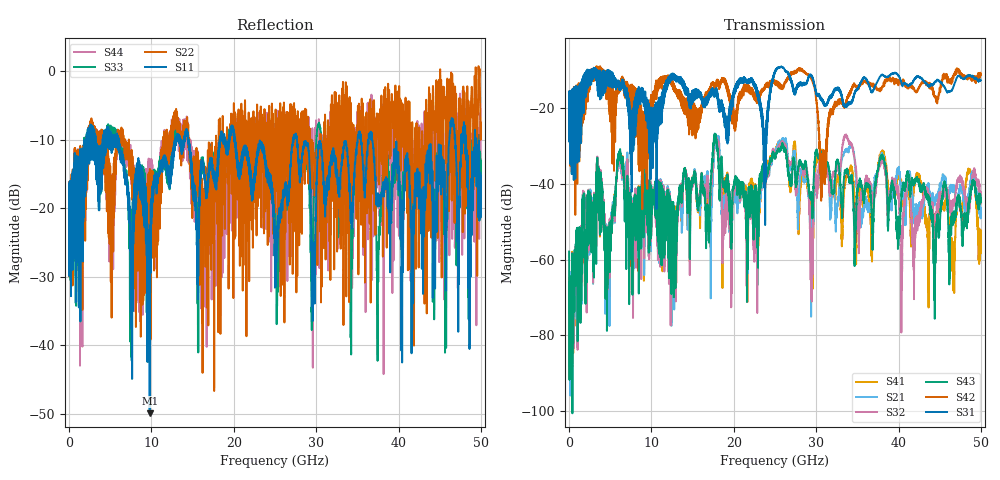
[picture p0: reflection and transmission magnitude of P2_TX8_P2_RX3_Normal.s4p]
!Keysight Technologies,N5225B,MY57041031,A.13.20.10
!Date: Friday, May 31, 2019 11:31:29
!Correction: S11(Full 4 Port(1,2,3,4))
!S12(Full 4 Port(1,2,3,4))
!S13(Full 4 Port(1,2,3,4))
!S14(Full 4 Port(1,2,3,4))
!S21(Full 4 Port(1,2,3,4))
!S22(Full 4 Port(1,2,3,4))
!S23(Full 4 Port(1,2,3,4))
!S24(Full 4 Port(1,2,3,4))
!S31(Full 4 Port(1,2,3,4))
!S32(Full 4 Port(1,2,3,4))
!S33(Full 4 Port(1,2,3,4))
!S34(Full 4 Port(1,2,3,4))
!S41(Full 4 Port(1,2,3,4))
!S42(Full 4 Port(1,2,3,4))
!S43(Full 4 Port(1,2,3,4))
!S44(Full 4 Port(1,2,3,4))
!S4P File: Measurements: <S11,S12,S13,S14>,
!<S21,S22,S23,S24>,
!<S31,S32,S33,S34>,
!<S41,S42,S43,S44>:
# Hz S  dB  R 50.0
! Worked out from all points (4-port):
!   5000 points, 10 MHz to 50 GHz, reference 50 ohm
!   strongest paths, dB at 10 MHz, 12.51 GHz, 25.01 GHz, 37.51 GHz, 50 GHz:
!     S31: -19.4, -11.7, -10.3, -12.8, -12.8
!     S42: -19.4, -14.3, -13.1, -15.4, -11.4
!     S43: -57.9, -45.1, -33.0, -36.5, -44.9
!     S32: -65.9, -45.2, -32.9, -36.8, -45.2
!     S21: -63.3, -46.2, -32.2, -37.2, -47.5
!     S41: -64.6, -45.6, -31.9, -36.0, -53.7
!   lowest |S11| = -49.9 dB at 9.79 GHz (marker M1), VSWR 1.01, Z = 50 - j0.317 ohm
!   |S11| at or under -10 dB: 20.17 GHz to 27.18 GHz (7.01 GHz wide, 29.6 % of centre); 27.67 GHz to 35.04 GHz (7.369 GHz wide, 23.5 % of centre); 36.79 GHz to 46.16 GHz (9.376 GHz wide, 22.6 % of centre)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
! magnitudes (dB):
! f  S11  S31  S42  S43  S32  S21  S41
! 10 MHz  -19.6  -19.4  -19.4  -57.9  -65.9  -63.3  -64.6
! 3.57 GHz  -19.0  -17.0  -12.5  -37.3  -36.5  -36.7  -37.4
! 9.79 GHz  -49.9  -26.2  -22.5  -46.0  -45.0  -45.5  -46.4
! 28.09 GHz  -14.3  -14.0  -9.9  -34.2  -34.9  -37.9  -40.2
! 30.79 GHz  -14.3  -18.0  -31.9  -32.5  -33.2  -35.1  -32.2
! 38.03 GHz  -17.9  -11.3  -14.4  -32.3  -33.9  -32.4  -31.4
! 50 GHz  -15.2  -12.8  -11.4  -44.9  -45.2  -47.5  -53.7
